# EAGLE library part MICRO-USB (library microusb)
Micro USB B connector
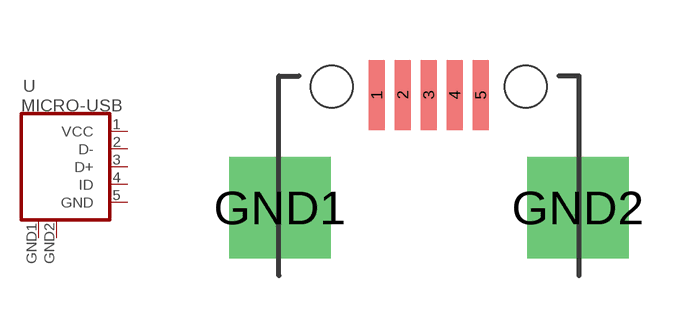
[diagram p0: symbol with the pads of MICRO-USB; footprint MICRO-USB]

Designator prefix -

## MICRO-USB  [MICRO-USB]
1  VCC  pwr
2  D-
3  D+
4  ID
5  GND  pwr
GND1  GND  pwr
GND2  GND  pwr

## Footprint MICRO-USB (pad centres in mm)
smd 0.4 x 1.75: 1 -1.3,4.525; 2 -0.65,4.525; 3 0,4.525; 4 0.65,4.525; 5 1.3,4.525
drill 1.2 pad 2.54 square: GND1 -3.725,1.7; GND2 3.725,1.7
hole 1.05 at -2.425,4.73
hole 1.05 at 2.425,4.73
